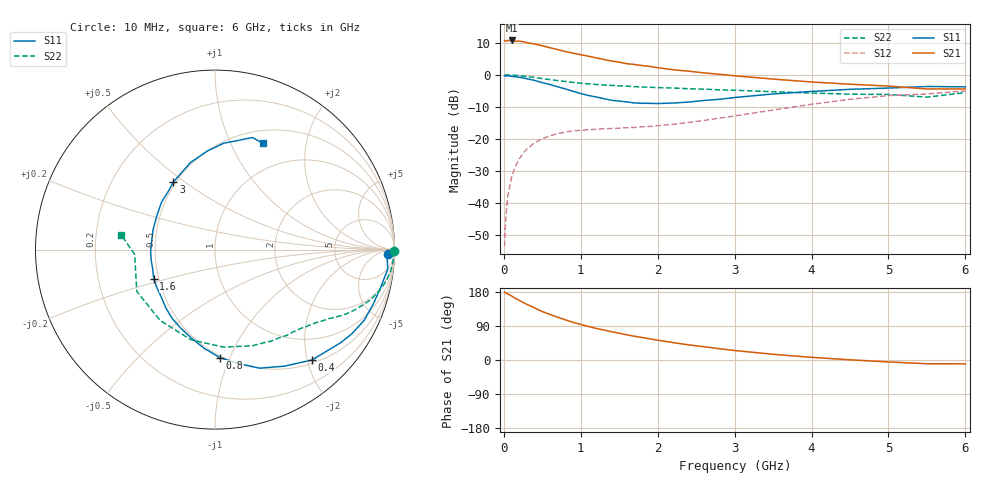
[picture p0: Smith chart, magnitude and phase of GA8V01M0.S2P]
! Infineon Technologies  Discrete & RF Semiconductors
! BF775
! Si NPN RF Bipolar Junction Transistor in SOT23
! VCE = 8 V  IC = 1 mA
! Common Emitter S-Parameters:  May  1996
# GHz  S  MA  R  50
!  f  S11  S21  S12  S22
! GHz  MAG  ANG  MAG  ANG  MAG  ANG  MAG  ANG
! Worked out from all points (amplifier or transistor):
!   36 points, 10 MHz to 6 GHz, reference 50 ohm
!   highest |S21| = 10.8 dB at 100 MHz (marker M1)
!   |S21| within 3 dB of that: start of sweep to 724.4 MHz
!   unconditionally stable (mu >= 1): 1.462 GHz to 3.485 GHz; 5.366 GHz to 5.87 GHz
!   at 250 MHz: K = 0.19, MSG = 17.4 dB, |S12| = -24.5 dB
!   at 1.4 GHz: K = 0.97, MSG = 10.6 dB, |S12| = -16.8 dB
!   at 6 GHz: K = 0.99, MSG = 0.3 dB, |S12| = -5.0 dB
!   S11 on the Smith chart (normalised r, x): 10 MHz: 40, -25; 400 MHz: 0.56, -2.09; 800 MHz: 0.49, -0.92; 1.6 GHz: 0.47, -0.18; 3 GHz: 0.48, +0.45; 6 GHz: 0.65, +1.34
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0.01  0.9649 -1.3  3.45 179.1  0.0021 92.0  0.9999 -0.4
0.02  0.9593 -2.5  3.371 177.6  0.0049 84.5  0.9973 -1.0
0.05  0.9688 -6.4  3.435 174.5  0.0124 86.8  0.9961 -2.4
0.1  0.9468 -12.9  3.45 169.0  0.025 81.9  0.991 -5.0
0.15  0.9325 -19.0  3.359 162.7  0.037 77.8  0.9838 -7.5
0.25  0.8954 -31.6  3.299 152.0  0.0595 70.8  0.9586 -12.1
0.4  0.8186 -48.7  3.044 137.5  0.0867 61.3  0.9114 -17.8
0.5  0.7561 -59.2  2.847 127.8  0.1008 55.9  0.8733 -21.1
0.6  0.7061 -69.3  2.654 120.2  0.1117 51.4  0.8426 -23.8
0.8  0.603 -87.3  2.312 105.9  0.1278 44.4  0.7871 -28.0
0.9  0.5534 -96.3  2.186 99.3  0.133 42.2  0.7623 -29.8
1.1  0.4759 -114.0  1.956 88.5  0.139 39.0  0.723 -33.1
1.3  0.4252 -130.0  1.739 79.1  0.1439 37.4  0.6941 -35.9
1.6  0.3779 -154.5  1.494 66.3  0.1494 37.3  0.6651 -40.1
1.9  0.3587 -178.6  1.352 55.6  0.1564 40.4  0.6397 -44.9
2.2  0.3626 161.7  1.202 45.9  0.1686 43.1  0.6228 -50.1
3  0.4423 121.6  0.967 25.0  0.2278 48.7  0.5748 -68.8
3.5  0.5033 105.9  0.859 15.1  0.2823 47.7  0.5456 -84.8
4.5  0.5944 85.4  0.714 0.5  0.4151 37.2  0.4991 -127.8
5  0.6221 77.9  0.668 -5.1  0.4747 28.9  0.4939 -151.9
5.5  0.658 71.6  0.602 -9.9  0.504 19.2  0.4485 -176.6
6  0.6498 65.5  0.603 -10.1  0.5598 14.1  0.5279 171.2
